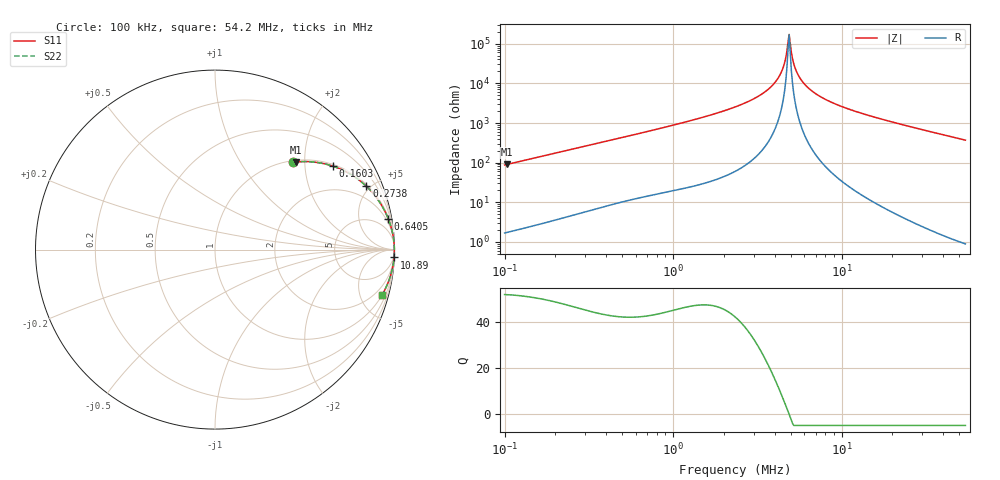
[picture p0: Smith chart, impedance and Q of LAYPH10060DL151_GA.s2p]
! LAYPH10060DL151_GA  S-PARAMETER MODEL  ( General Type )
! Model Generated by TAIYO YUDEN Corporation (http://www.ty-top.com)
! Version 3.0
! TAIYO YUDEN Control No. 180828NI43SB-FBB
! Copyright(c) 2017 TAIYO YUDEN CO.,LTD. All Rights Reserved.
! Product Description (link to TY-COMPAS)
! https://ds.yuden.co.jp/TYCOMPAS/or/detail?pn=LAYPH10060DL151MGA&u=M
! Products Name : Inductors
! Characteristics :
!  Inductance : 150 uH , SRF(min) : -Hz , DC Resistance(max) : 0.295 Ohm
!  Rated Current : Saturation :1.2 A , Temp Rise : 0.72 A (25 degC)
!  Case Size : 10.1 x 10.0 / 0.398 x 0.394 [mm/inch] , Thickness : 6 / 0.236 [mm/inch]
!  (Conditions: Temperature = 25 degC , DC Bias Current/Voltage = 0A / 0V)
! External Node Assignments :
!  1  o---GGG---o  2
! GND o---------o GND
! Frequency Range : 0.1MHz  -  54.20166MHz  [ 402 STEP ]
# MHz S RI R 50
! Freq[MHz].  S11 Real  S11 Imag  S21 Real  S21 Imag  S12 Real  S12 Imag  S22 Real  S22 Imag
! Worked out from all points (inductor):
!   401 points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, 100 kHz to 54.2 MHz, reference 50 ohm
!   read as one part in series: L = 139 uH near 103.2 kHz
!   highest Q = 51.9 at 103.2 kHz (marker M1), where L = 139 uH
!   self-resonance near 4.802 MHz
!   S11 on the Smith chart (normalised r, x): 100 kHz: 1.03, +1.75; 160.3 kHz: 1.06, +2.79; 273.8 kHz: 1.10, +4.74; 640.5 kHz: 1, +11; 10.89 MHz: 2, -46; 54.2 MHz: 1.02, -7.39
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0.1  0.4339 0.4861  0.5661 -0.4861  0.5661 -0.4861  0.4339 0.4861
0.103198  0.449 0.4879  0.551 -0.4879  0.551 -0.4879  0.449 0.4879
0.160343  0.6574 0.4647  0.3426 -0.4647  0.3426 -0.4647  0.6574 0.4647
0.273805  0.8436 0.3525  0.1564 -0.3525  0.1564 -0.3525  0.8436 0.3525
0.287043  0.8552 0.3411  0.1448 -0.3411  0.1448 -0.3411  0.8552 0.3411
0.640522  0.9647 0.1732  0.0353 -0.1732  0.0353 -0.1732  0.9647 0.1732
0.823937  0.978 0.1356  0.022 -0.1356  0.022 -0.1356  0.978 0.1356
2.328125  0.9975 0.0394  0.00249 -0.0394  0.00249 -0.0394  0.9975 0.0394
3.239977  0.9989 0.0205  0.00114 -0.0205  0.00114 -0.0205  0.9989 0.0205
3.975551  0.9993 0.01  0.000735 -0.01  0.000735 -0.01  0.9993 0.01
4.438565  0.9994 0.00456  0.000624 -0.00456  0.000624 -0.00456  0.9994 0.00456
4.580497  0.9994 0.00301  0.000604 -0.00301  0.000604 -0.00301  0.9994 0.00301
4.726969  0.9994 0.00147  0.00059 -0.00147  0.00059 -0.00147  0.9994 0.00147
4.878123  0.9994 -7.09e-05  0.00058 7.09e-05  0.00058 7.09e-05  0.9994 -7.09e-05
5.034112  0.9994 -0.00161  0.000576 0.00161  0.000576 0.00161  0.9994 -0.00161
5.277496  0.9994 -0.00393  0.00058 0.00393  0.00058 0.00393  0.9994 -0.00393
5.532648  0.9994 -0.00625  0.000596 0.00625  0.000596 0.00625  0.9994 -0.00625
5.985607  0.9994 -0.0102  0.000648 0.0102  0.000648 0.0102  0.9994 -0.0102
6.682722  0.9992 -0.0157  0.000778 0.0157  0.000778 0.0157  0.9992 -0.0157
10.88527  0.9976 -0.0437  0.00241 0.0437  0.00241 0.0437  0.9976 -0.0437
19.18229  0.9914 -0.0895  0.00858 0.0895  0.00858 0.0895  0.9914 -0.0895
54.20166  0.9313 -0.2518  0.0687 0.2518  0.0687 0.2518  0.9313 -0.2518
